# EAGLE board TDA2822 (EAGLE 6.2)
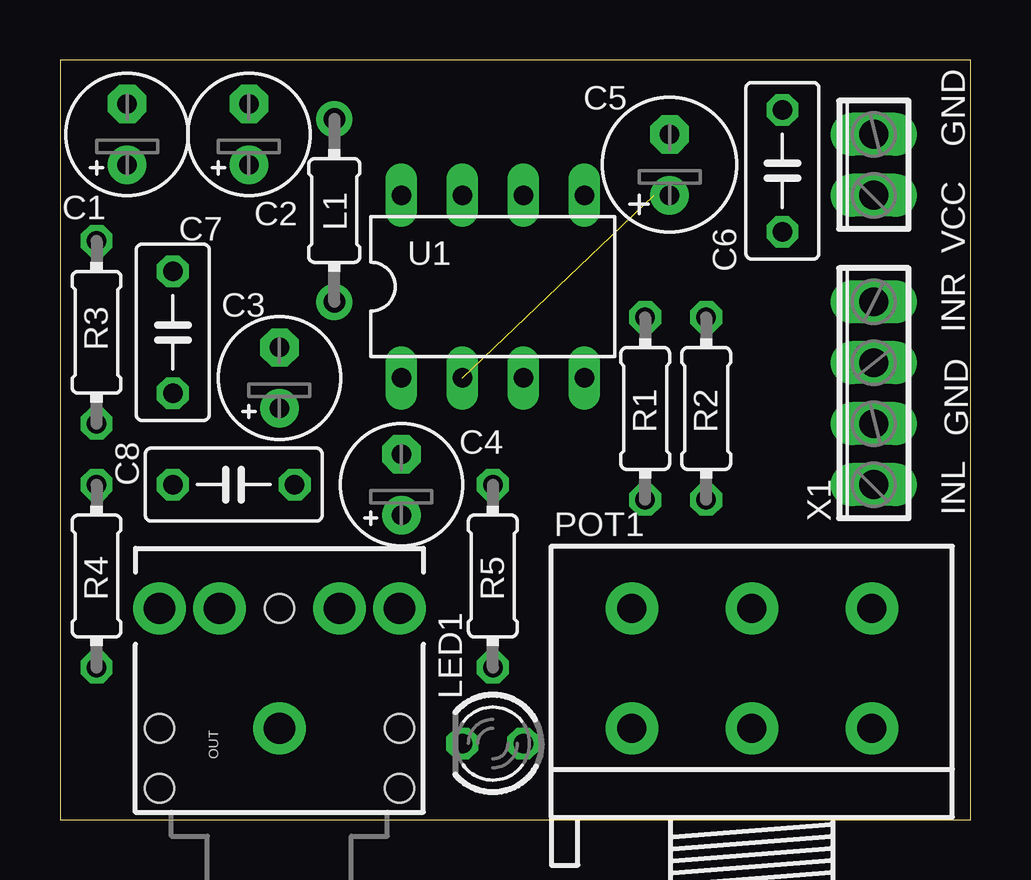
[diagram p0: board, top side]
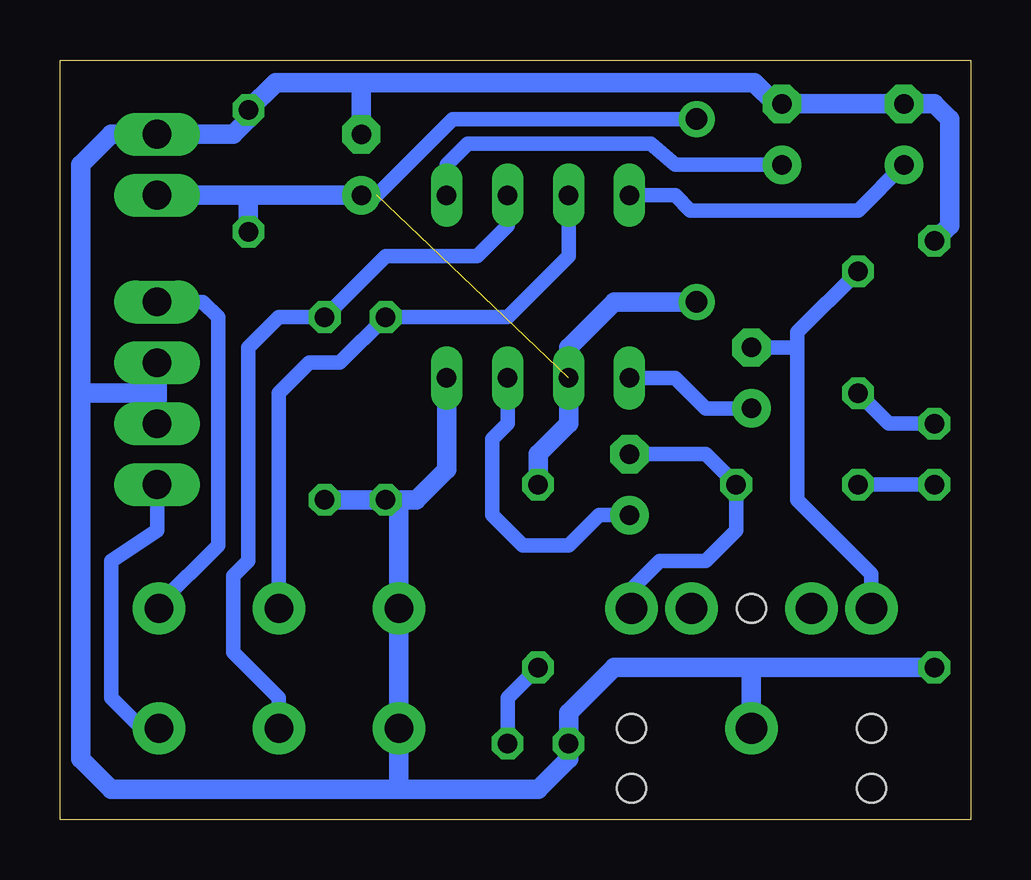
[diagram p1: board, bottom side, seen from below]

Size 37.95 x 31.67 mm. Coordinates in mm from the lower left corner, seen from the top.
Outline: 0,0 37.95,0 37.95,31.67 0,31.67 0,0
Copper layers (1*16): Top 0.035mm / dielectric 1.5mm / Bottom 0.035mm
Design rules: minimum track width 10mil, minimum drill 24mil, track to track 8mil, track to pad 8mil, pad to pad 8mil, via to via 8mil, smd to smd 8mil, copper to edge 40mil, drill to drill 8mil, minimum pad ring 10mil, minimum via ring 8mil, stop-mask expansion 4mil, vias tented up to drill 0mil, thermal gap 10mil

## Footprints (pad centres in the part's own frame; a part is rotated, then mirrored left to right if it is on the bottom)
E2,5-5 = drill 0.813 pad 1.6: + -1.27,0 | drill 0.813 pad 1.6 octagon: - 1.27,0
E2,5-6 = drill 0.813 pad 1.6: + -1.27,0 | drill 0.813 pad 1.6 octagon: - 1.27,0
C050-030X075 = drill 0.813 octagon: 1 -2.54,0; 2 2.54,0
TFI0204 = drill 0.9 pad 1.5: 1 -3.81,0; 2 3.81,0
LED3MM = drill 0.813 octagon: A -1.27,0; K 1.27,0
AUDIO-JACK = drill 1.3 pad 2.184: 1 0,0; 2 5,5; 3 5,2.5; 4 5,-2.5; 5 5,-5 | hole 1.2: 0,5; -2.5,5; -2.5,-5; 0,-5; 5,0
3RP/1610G = drill 1.2 pad 2.184: 1-1 -5,0; 1-2 0,0; 1-3 5,0; 2-1 -5,5; 2-2 0,5; 2-3 5,5
0204/7 = drill 0.813 octagon: 1 -3.81,0; 2 3.81,0
DIL8 = drill 0.813 long: 1 -3.81,-3.81; 2 -1.27,-3.81; 3 1.27,-3.81; 4 3.81,-3.81; 5 3.81,3.81; 6 1.27,3.81; 7 -1.27,3.81; 8 -3.81,3.81
2POL254 = drill 1.2 long: 1 -1.27,0; 2 1.27,0
4POL254 = drill 1.2 long: 1 -3.81,0; 2 -1.27,0; 3 1.27,0; 4 3.81,0

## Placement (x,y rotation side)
C1  100uF  [E2,5-5]  2.79,28.57 90 top
C2  [E2,5-5]  7.87,28.57 90 top
C3  100uF  [E2,5-5]  9.14,18.41 90 top
C4  [E2,5-5]  14.22,13.97 90 top
C5  [E2,5-6]  25.4,27.3 90 top
C6  [C050-030X075]  30.1,27.05 90 top
C7  100nF  [C050-030X075]  4.7,20.32 270 top
C8  [C050-030X075]  7.24,13.97 180 top
L1  [TFI0204]  11.43,25.4 270 top
LED1  [LED3MM]  18.03,3.17 180 top
OUT  AUDIO-JACKPTH  [AUDIO-JACK]  9.14,3.81 90 top
POT1  [3RP/1610G]  28.83,3.81 0 top
R1  10k  [0204/7]  24.38,17.14 90 top
R2  [0204/7]  26.92,17.14 90 top
R3  4,7  [0204/7]  1.52,20.32 270 top
R4  [0204/7]  1.52,10.16 90 top
R5  [0204/7]  18.03,10.16 90 top
U1  TDA2822M  [DIL8]  18.03,22.23 0 top
VCC  [2POL254]  33.91,27.3 90 top
X1  [4POL254]  33.91,17.78 90 top

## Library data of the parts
C1-C8 L1 R1-R5 = rcl
LED1 = led
OUT = moja
POT1 = pot
U1 = TDA2822M
VCC X1 = con-phoenix-254; OC_FARNELL: unknown; OC_NEWARK: unknown

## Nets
GND: C1.- C2.- C5.- C6.2 LED1.K OUT.1 POT1.1-1 POT1.2-1 R1.1 R2.1 R3.1 R4.1 U1.4 VCC.2 X1.2 X1.3
N$1: C1.+ U1.8
N$2: C2.+ U1.5
N$3: C3.+ U1.1
N$4: C4.+ U1.3
N$5: C3.- C7.1 OUT.2
N$6: C4.- C8.1 OUT.5
N$7: C7.2 R3.2
N$8: C8.2 R4.2
N$9: POT1.2-2 R1.2 U1.7
N$10: POT1.1-2 R2.2 U1.6
N$11: POT1.2-3 X1.4
N$13: L1.2 R5.2
N$14: LED1.A R5.1
N$15: POT1.1-3 X1.1
VCC: C5.+ C6.1 L1.1 U1.2 VCC.1

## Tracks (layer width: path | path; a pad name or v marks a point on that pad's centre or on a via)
GND
  Bottom 0.813: R3.1 0.89,24.77 0.89,29.21 1.52,29.84 C1.- C2.- 8.13,29.84 9.02,30.73 25.27,30.73 | U1.4 21.84,14.61 23.11,13.34 23.75,13.34 | 23.75,13.34 R1.1 R2.1 | 23.75,13.34 23.83,13.26 POT1.2-1 POT1.1-1 23.83,1.35 23.75,1.27 | R4.1 9.14,6.35 | 9.14,6.35 14.86,6.35 16.76,4.45 LED1.K 16.76,2.54 18.03,1.27 23.75,1.27 | OUT.1 9.14,6.35 | X1.3 X1.2 33.91,17.78 37.08,17.78 | 37.08,17.78 37.08,27.3 35.81,28.57 VCC.2 30.73,28.57 30.1,29.21 C6.2 28.96,30.73 25.27,30.73 | 37.08,17.78 37.08,2.54 35.81,1.27 23.75,1.27 | C5.- 25.4,30.61 25.27,30.73
N$1
  Bottom 0.61: C1.+ 4.7,25.4 11.68,25.4 12.32,26.04 U1.8
N$2
  Bottom 0.61: U1.5 21.84,27.3 20.95,28.19 13.33,28.19 12.32,27.3 C2.+
N$3
  Bottom 0.61: U1.1 12.32,18.41 11.05,17.14 C3.+
N$4
  Bottom 0.61: C4.+ 15.49,12.7 16.76,11.43 18.67,11.43 19.94,12.7 19.94,15.88 19.3,16.51 U1.3
N$5
  Bottom 0.61: C3.- 7.24,19.68 | 7.24,19.68 7.24,20.32 C7.1 | OUT.2 4.14,10.24 7.24,13.34 7.24,19.68
N$6
  Bottom 0.61: C4.- 11.05,15.24 C8.1 9.78,12.06 11.05,10.79 12.95,10.79 14.14,9.61 OUT.5
N$7
  Bottom 0.61: R3.2 3.43,16.51 C7.2
N$8
  Bottom 0.61: R4.2 C8.2
N$9
  Bottom 0.61: U1.7 16.76,23.5 19.3,20.95 R1.2 26.29,19.05 27.56,19.05 28.83,17.78 POT1.2-2
N$10
  Bottom 0.61: U1.6 19.3,24.77 20.57,23.5 24.38,23.5 R2.2 28.83,20.95 30.1,19.68 30.1,10.79 30.73,10.16 30.73,6.99 28.83,5.08 POT1.1-2
N$11
  Bottom 0.61: 33.83,8.97 31.37,11.43 31.37,20.95 32,21.59 X1.4
  Bottom 0.813: POT1.2-3 33.83,8.97
N$13
  Bottom 0.813: R5.2 18.03,15.24 16.76,16.51 16.76,19.68 14.86,21.59 L1.2
N$14
  Bottom 0.61: R5.1 19.3,5.08 LED1.A
N$15
  Bottom 0.61: POT1.1-3 34.54,3.81 35.81,5.08 35.81,10.79 33.91,12.06 X1.1
VCC  (1 unrouted)
  Bottom 0.61: L1.1 21.59,29.21 24.77,26.04 C5.+
  Bottom 0.813: C5.+ 30.1,26.04 | 30.1,26.04 VCC.1 | C6.1 30.1,26.04

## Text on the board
tNames: GND | INR | GND | INL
